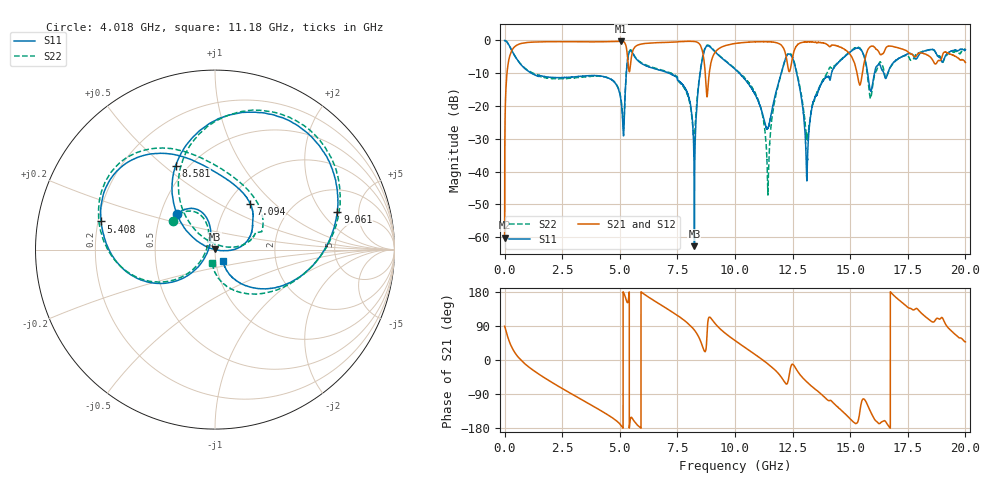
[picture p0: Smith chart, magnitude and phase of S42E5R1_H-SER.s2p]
! Created Sat Jan  9 20:26:59 2021
# hz S ma R 50
! 2 Port Network Data from SP1.SP block
! freq  magS11  angS11  magS21  angS21  magS12  angS12  magS22  angS22
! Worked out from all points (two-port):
!   20001 points, 300 kHz to 20 GHz, reference 50 ohm
!   highest |S21| = -0.24 dB at 5.042 GHz (marker M1); lowest = -60.2 dB at 300 kHz (marker M2)
!   |S21| within 3 dB of the highest: 301.7 MHz to 5.308 GHz (5.006 GHz wide, 178 % of centre); 5.561 GHz to 8.586 GHz (3.025 GHz wide, 42.8 % of centre)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
!   lowest |S11| = -62.8 dB at 8.239 GHz (marker M3), VSWR 1.00, Z = 50 + j0.0679 ohm
!   |S11| at or under -10 dB: 1.164 GHz to 5.283 GHz (4.119 GHz wide, 128 % of centre); 10.19 GHz to 12 GHz (1.814 GHz wide, 16.4 % of centre); 12.68 GHz to 14.19 GHz (1.511 GHz wide, 11.2 % of centre)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
!   |S22| runs from -47.2 to 0.0 dB; largest |S21 - S12| = 0.018
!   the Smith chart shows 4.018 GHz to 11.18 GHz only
!   S11 on the Smith chart (normalised r, x): 4.018 GHz: 0.61, +0.26; 5.408 GHz: 0.21, +0.12; 7.094 GHz: 1.27, +0.71; 8.581 GHz: 0.43, +0.55; 9.061 GHz: 3.40, +2.88; 11.18 GHz: 1.09, -0.14
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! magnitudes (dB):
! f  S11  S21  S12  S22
! 300 kHz  0.0  -60.2  -59.9  0.0
! 116.3 MHz  -0.6  -9.1  -9.1  -0.6
! 347.3 MHz  -3.5  -2.7  -2.6  -3.5
! 3.334 GHz  -10.9  -0.4  -0.4  -11.2
! 4.018 GHz  -10.7  -0.4  -0.4  -10.9
! 5.042 GHz  -17.8  -0.2  -0.3  -17.5
! 5.408 GHz  -3.7  -9.5  -9.5  -3.4
! 6.667 GHz  -8.9  -0.7  -0.7  -8.7
! 7.094 GHz  -9.9  -0.6  -0.6  -9.7
! 8.239 GHz  -62.8  -0.3  -0.3  -29.9
! 8.581 GHz  -5.7  -3.1  -3.1  -5.5
! 9.061 GHz  -2.9  -4.5  -4.5  -2.8
! 10 GHz  -8.7  -0.9  -0.9  -8.6
! 11.18 GHz  -22.1  -0.4  -0.4  -22.4
! 11.44 GHz  -26.5  -0.4  -0.4  -43.5
! 12.35 GHz  -4.1  -9.5  -9.4  -3.9
! 13.1 GHz  -40.4  -0.5  -0.5  -29.3
! 13.33 GHz  -20.7  -0.5  -0.5  -20.5
! 15.21 GHz  -2.5  -7.4  -7.5  -2.3
! 15.88 GHz  -15.4  -1.8  -1.9  -17.6
! 16.67 GHz  -9.3  -1.7  -1.8  -9.4
! 20 GHz  -2.8  -6.7  -6.7  -2.6
